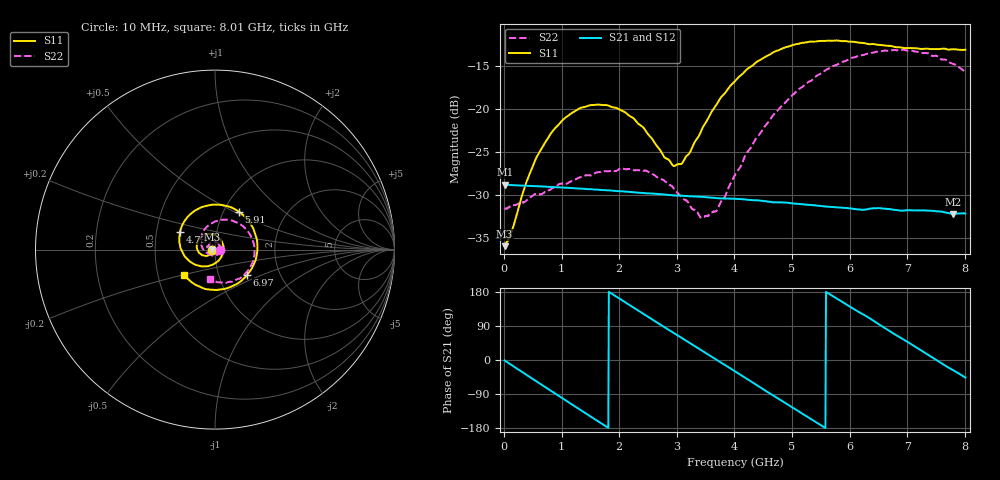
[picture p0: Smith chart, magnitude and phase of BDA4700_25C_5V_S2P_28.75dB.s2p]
!Agilent Technologies,E5071B,MY42404982,A.09.10
!Date: Mon Oct 20 13:41:03 2025
!Data & Calibration Information:
!Freq	S11:SOLT2(ON)	S21:SOLT2(ON)	S12:SOLT2(ON)	S22:SOLT2(ON)
# Hz S RI R 50
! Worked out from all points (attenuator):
!   801 points, 10 MHz to 8.01 GHz, reference 50 ohm
!   highest |S21| = -28.82 dB at 20 MHz (marker M1); lowest = -32.2 dB at 7.79 GHz (marker M2)
!   lowest |S11| = -36.0 dB at 10 MHz (marker M3), VSWR 1.03, Z = 48.4 - j0.122 ohm
!   |S11| at or under -10 dB: start of sweep to end of sweep
!   |S22| runs from -32.7 to -13.1 dB; largest |S21 - S12| = 0.00029
!   S11 on the Smith chart (normalised r, x): 10 MHz: 0.97, -0.00; 4.73 GHz: 0.66, +0.14; 5.91 GHz: 1.17, +0.53; 6.97 GHz: 1.37, -0.40; 8.01 GHz: 0.68, -0.20
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1e7  -0.0158 -0.00126  0.0362 -0.000744  0.0362 -0.00081  0.0262 -0.00079
2e7  -0.0162 -0.00197  0.0362 -0.00135  0.0362 -0.00147  0.0261 -0.00107
6e8  -0.0428 -0.0346  0.0177 -0.0307  0.0177 -0.0307  0.0127 -0.0291
1e9  -0.0817 -0.0238  -0.0058 -0.0343  -0.00586 -0.0344  -0.0146 -0.0338
1.35e9  -0.1017 0.0118  -0.0239 -0.0247  -0.0239 -0.0246  -0.036 -0.0179
2.07e9  -0.0453 0.086  -0.0301 0.0136  -0.0301 0.0136  -0.0305 0.033
2.68e9  0.0369 0.0466  -0.00372 0.0317  -0.00376 0.0317  0.0127 0.0375
2.93e9  0.0467 0.00523  0.00927 0.03  0.0093 0.03  0.0246 0.0249
3.06e9  0.0442 -0.0181  0.0154 0.0272  0.0153 0.0272  0.0273 0.0149
3.44e9  -0.000388 -0.0769  0.028 0.0126  0.0281 0.0126  0.0186 -0.0139
3.69e9  -0.0513 -0.0932  0.0302 0.000264  0.0302 0.000158  0.000656 -0.0254
4.01e9  -0.1248 -0.0759  0.0259 -0.0149  0.0259 -0.0149  -0.032 -0.0256
4.39e9  -0.1894 0.00112  0.0118 -0.027  0.0117 -0.027  -0.0683 0.00475
4.73e9  -0.1949 0.1002  -0.00434 -0.0282  -0.00428 -0.0283  -0.0792 0.0556
5.35e9  -0.06 0.2408  -0.0255 -0.0104  -0.0255 -0.0105  -0.0156 0.1476
5.91e9  0.1323 0.2122  -0.0229 0.0135  -0.0229 0.0134  0.109 0.1564
6.27e9  0.2154 0.1117  -0.0119 0.023  -0.0117 0.0231  0.1825 0.1018
6.68e9  0.2306 -0.0419  0.0056 0.0255  0.00567 0.0255  0.2197 0.000744
6.97e9  0.1798 -0.1398  0.0161 0.0199  0.0162 0.0199  0.2071 -0.0773
7.37e9  0.0507 -0.2198  0.0249 0.00576  0.0248 0.00575  0.1371 -0.1613
7.79e9  -0.1092 -0.1956  0.0219 -0.0108  0.0219 -0.0109  0.0233 -0.1828
8.01e9  -0.1712 -0.1423  0.0169 -0.0178  0.0169 -0.0179  -0.03 -0.1623
